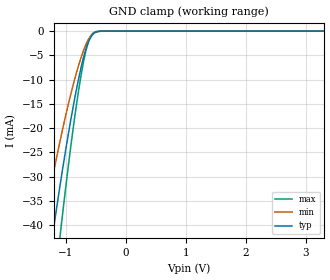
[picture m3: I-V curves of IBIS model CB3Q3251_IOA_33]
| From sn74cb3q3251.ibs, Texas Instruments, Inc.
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[Model]   CB3Q3251_IOA_33
Model_type  Terminator
| variable   typ   min   max
C_comp   2.33pF   1.82pF   2.77pF
| C_tri-state   2.33pF   1.82pF   2.77pF
[Temperature Range]   40   100   -40
| Ambient temperature   25   85   -40
[Voltage range]   3.3   3   3.6
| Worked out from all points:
|   GND clamp passes 1 mA (typ) near -0.57 V on its own axis
[GND Clamp]
| CB3Q3251_IOA_33
|   Voltage   I(typ)   I(min)   I(max)
-5.5V     -546.9mA   -436.2mA   -659.1mA
-1.39V    -57.48mA   -41.37mA   -76.9mA
-1.215V   -41.72mA   -29.83mA   -55.76mA
-1.195V   -40.01mA   -28.58mA   -53.44mA
-1.105V   -32.54mA   -23.18mA   -43.28mA
-1.08V    -30.54mA   -21.73mA   -40.54mA
-895mV    -16.78mA   -11.93mA   -21.68mA
-740mV    -7.209mA   -5.232mA   -8.708mA
-680mV    -4.328mA   -3.206mA   -4.842mA
-625mV    -2.318mA   -1.756mA   -2.24mA
-530mV    -464.7uA   -384.9uA   -271.2uA
3.3V      142.5pA    602.8pA    19.2pA
